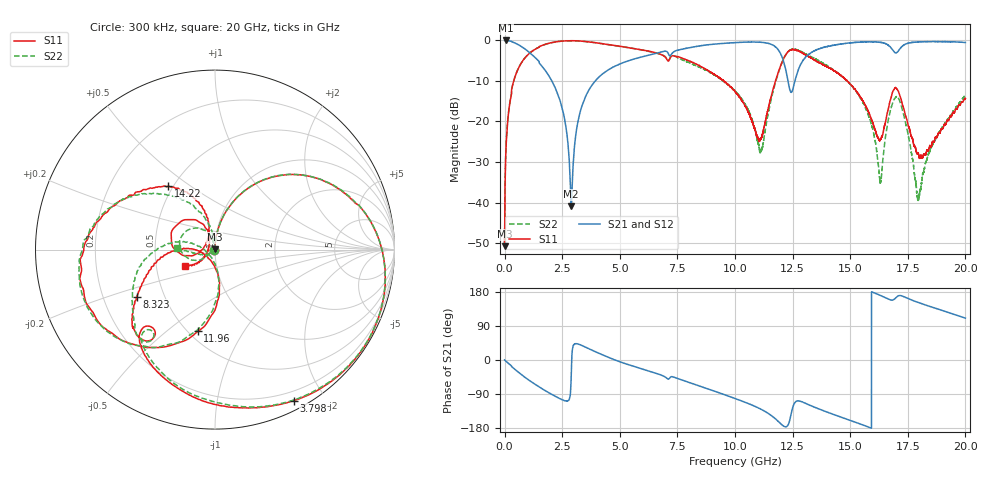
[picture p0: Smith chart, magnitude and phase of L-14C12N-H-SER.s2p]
!{L-14C12N}
!Johanson Technology Inc.
!www.johansontechnology.com
!Test Board Conditions:
!Substrate Type  RO4350B
!Substrate Thickness  20 mil
!Substrate Dk  3.66
!TL Type: GCPW
!TL Trace Width  36 mil
!TL Gap  12 mil
!Electrode orientation  Horizontal
!DUT TOPOLOGY	SERIES
!Mounting Pad LxW  26x36 mil
! Created Sun Jun 20 13:00:57 2021
# hz S ma R 50
! 2 Port Network Data from SP1.SP block
! freq  magS11  angS11  magS21  angS21  magS12  angS12  magS22  angS22
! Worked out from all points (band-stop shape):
!   20001 points, 300 kHz to 20 GHz, reference 50 ohm
!   highest |S21| = -0.01 dB at 48.3 MHz (marker M1); lowest = -41.0 dB at 2.894 GHz (marker M2)
!   |S21| within 3 dB of the highest: 7.299 GHz to 11.96 GHz (4.656 GHz wide, 48.4 % of centre); 13.3 GHz to 16.94 GHz (3.64 GHz wide, 24.1 % of centre)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
!   lowest |S11| = -50.8 dB at 1.3 MHz (marker M3), VSWR 1.01, Z = 49.7 + j0.116 ohm
!   |S11| at or under -10 dB: start of sweep to 397.1 MHz; 9.506 GHz to 11.76 GHz (2.252 GHz wide, 21.2 % of centre); 14.87 GHz to end of sweep
!   |S22| runs from -50.3 to -0.1 dB; largest |S21 - S12| = 0.015
!   S11 on the Smith chart (normalised r, x): 300 kHz: 0.99, -0.00; 3.798 GHz: 0.10, -1.64; 8.323 GHz: 0.35, -0.25; 11.96 GHz: 0.56, -0.65; 14.22 GHz: 0.47, +0.41; 20 GHz: 0.70, -0.14
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300000  0.004756 -161.0  0.9961 0.2  0.995 0.2  0.004662 -156.5
1300000  0.002893 156.3  0.9973 0.0  0.9973 -0.0  0.003063 153.2
4.83e7  0.0375 88.1  0.999 -2.6  0.998 -2.7  0.03799 88.1
2.263e8  0.168 77.7  0.9848 -12.0  0.9835 -12.0  0.1695 77.6
6.293e8  0.4706 55.2  0.8752 -33.8  0.8742 -33.9  0.4723 55.3
2.2863e9  0.9665 -11.0  0.2261 -98.6  0.2263 -98.6  0.9638 -10.7
2.8943e9  0.992 -32.5  0.008964 -35.1  0.009004 -35.4  0.9899 -32.0
3.3343e9  0.9802 -47.8  0.1484 38.8  0.1488 38.9  0.9778 -46.9
3.7983e9  0.9486 -62.5  0.2817 25.9  0.282 25.8  0.9485 -61.4
6.6673e9  0.6901 -126.1  0.7044 -37.0  0.7053 -36.8  0.6869 -124.3
8.3233e9  0.5098 -149.0  0.8428 -65.9  0.8452 -65.6  0.488 -158.1
1.00003e10  0.2349 -177.8  0.9382 -101.6  0.9396 -101.7  0.2387 170.6
1.11293e10  0.06257 -118.8  0.9475 -130.1  0.9464 -130.0  0.04351 -136.7
1.19563e10  0.4653 -101.9  0.7064 -166.5  0.7114 -166.6  0.4595 -102.4
1.24443e10  0.7648 -151.8  0.2284 -140.3  0.2318 -141.4  0.7729 -150.4
1.33343e10  0.5994 153.4  0.7163 -121.7  0.7118 -122.0  0.6203 157.0
1.42243e10  0.4381 126.4  0.8653 -142.6  0.8615 -142.8  0.4405 135.1
1.62973e10  0.05871 154.7  0.9483 170.8  0.9455 170.9  0.01787 152.9
1.66673e10  0.1474 -166.7  0.869 160.3  0.866 160.5  0.1099 -147.0
1.71553e10  0.2066 126.0  0.7865 170.1  0.7824 170.4  0.1763 139.1
1.79743e10  0.03841 151.5  0.9579 151.3  0.9571 151.1  0.01165 166.2
2e10  0.1914 -150.7  0.9418 110.4  0.9338 110.2  0.2122 177.9
